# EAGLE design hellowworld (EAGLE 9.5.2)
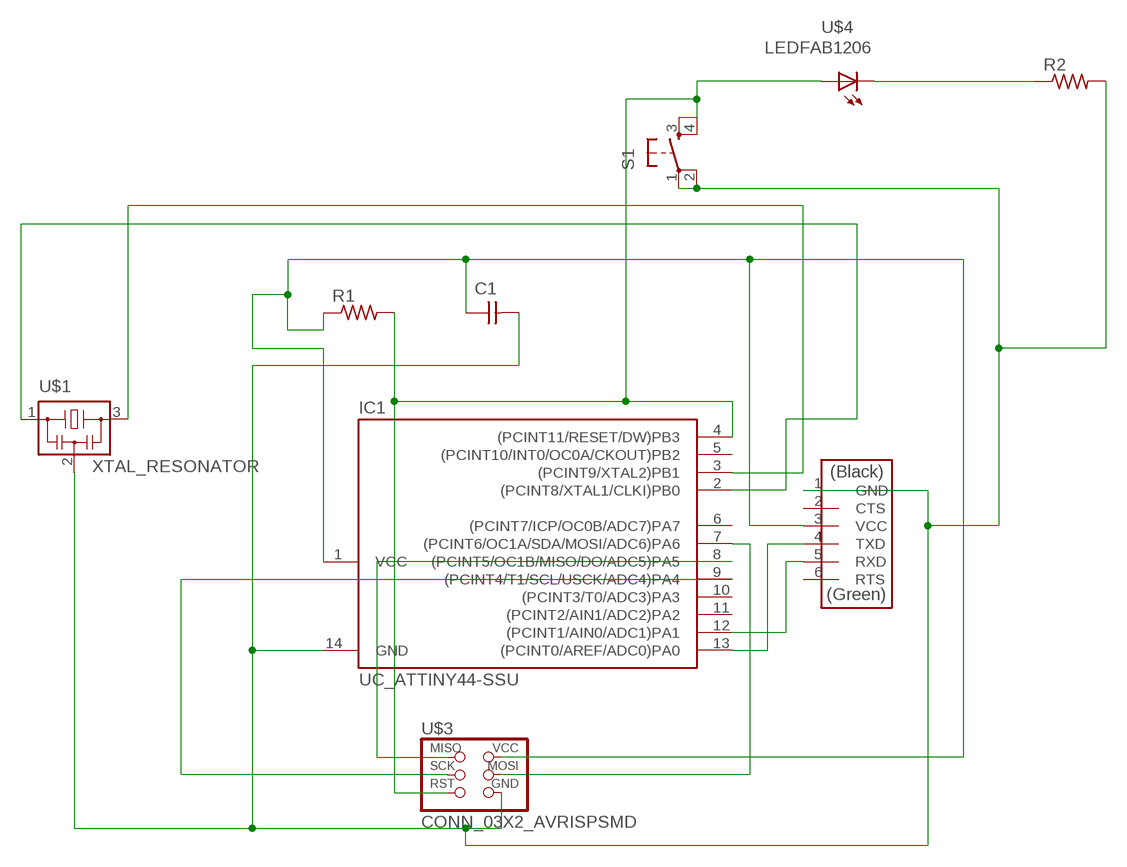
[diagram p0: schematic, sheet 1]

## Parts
C1  CAP_UNPOLARIZEDFAB  [C1206FAB]
IC1  UC_ATTINY44-SSU  [SOIC14]
R1  R1206FAB  [R1206FAB]
R2  R1206FAB  [R1206FAB]
S1  SW_SWITCH_TACTILE_6MM6MM_SWITCH  [6MM_SWITCH]
U$1  XTAL_RESONATOR  [EFOBM]
U$2  CONN_06_FTDI-SMD-HEADER  [1X06SMD]
U$3  CONN_03X2_AVRISPSMD  [2X03SMD]
U$4  LEDFAB1206  [LED1206FAB]

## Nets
N$1: IC1.13((PCINT0/AREF/ADC0)PA0) U$2.4(TXD)
N$2: C1.2 IC1.14(GND) R2.2 S1.1(P) S1.2(P1) U$1.2 U$2.1(GND) U$3.6(GND)
N$3: IC1.7((PCINT6/OC1A/SDA/MOSI/ADC6)PA6) U$3.4(MOSI)
N$4: IC1.8((PCINT5/OC1B/MISO/DO/ADC5)PA5) U$3.1(MISO)
N$5: IC1.9((PCINT4/T1/SCL/USCK/ADC4)PA4) U$3.3(SCK)
N$6: C1.1 IC1.1(VCC) R1.1 U$2.3(VCC) U$3.2(VCC)
N$7: IC1.2((PCINT8/XTAL1/CLKI)PB0) U$1.1
N$8: IC1.3((PCINT9/XTAL2)PB1) U$1.3
N$9: IC1.12((PCINT1/AIN0/ADC1)PA1) U$2.5(RXD)
N$10: R2.1 U$4.2(C)
N$11: IC1.4((PCINT11/RESET/DW)PB3) R1.2 S1.3(S) S1.4(S1) U$3.5(RST) U$4.1(A)
Unconnected: IC1.5((PCINT10/INT0/OC0A/CKOUT)PB2) IC1.6((PCINT7/ICP/OC0B/ADC7)PA7) IC1.10((PCINT3/T0/ADC3)PA3) IC1.11((PCINT2/AIN1/ADC2)PA2) U$2.2(CTS) U$2.6(RTS)

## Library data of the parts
C1 = eagle_fab:CAP_UNPOLARIZED
IC1 = eagle_fab:UC_ATTINY44
R1 R2 = eagle_fab:R: Resistor (US Symbol)
S1 = eagle_fab:SW_SWITCH_TACTILE_6MM: OMRON SWITCH
U$1 = eagle_fab:XTAL_RESONATOR
U$2 = eagle_fab:CONN_06_FTDI-SMD-HEADER
U$3 = eagle_fab:CONN_03X2_AVRISP
U$4 = eagle_fab:LED: LED

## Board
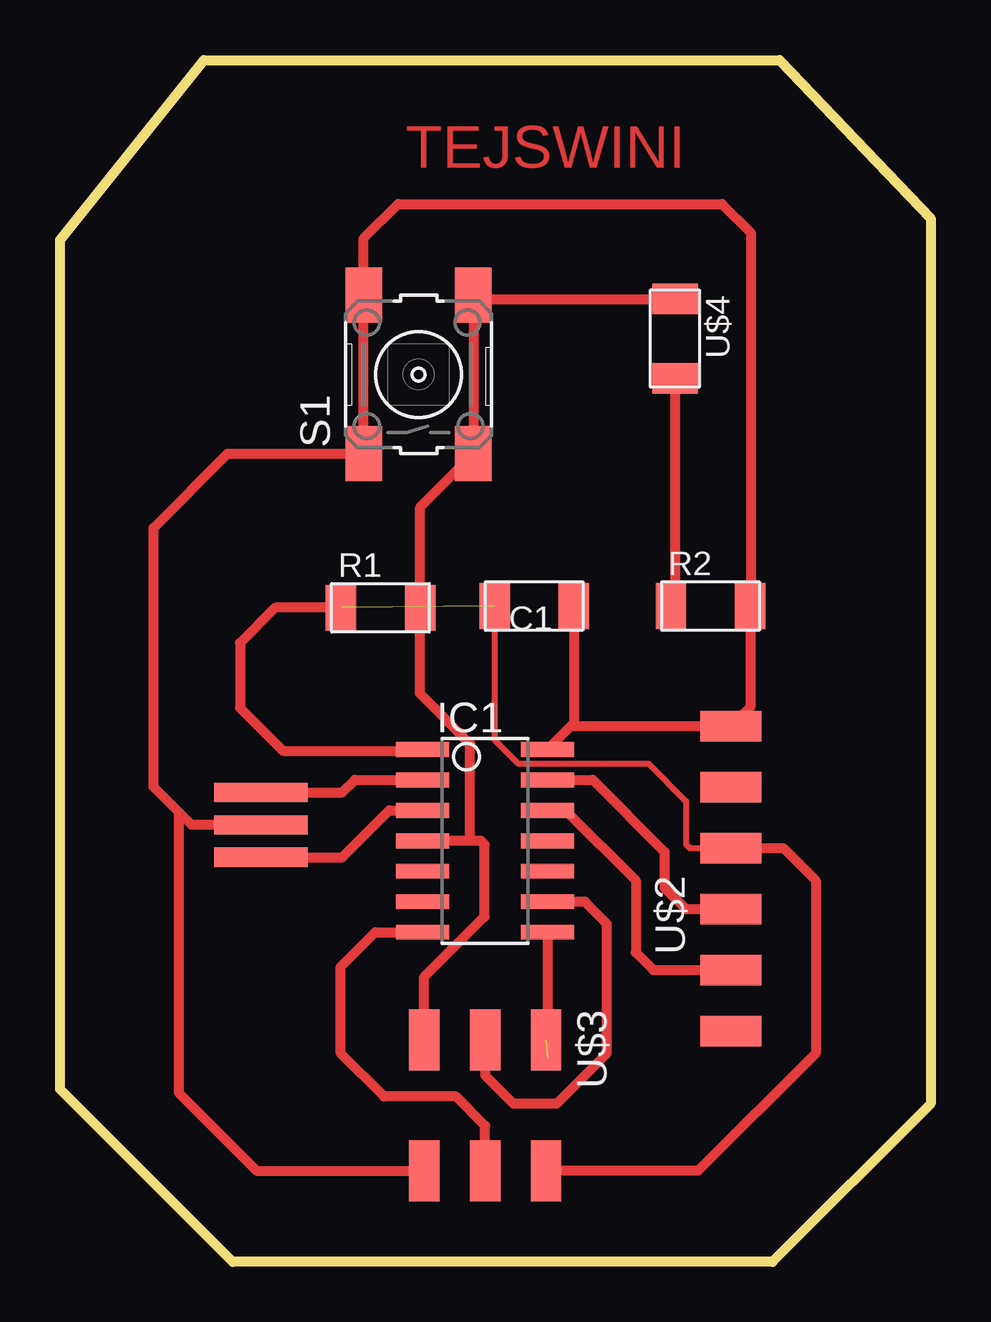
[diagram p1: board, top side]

Size 36.3 x 50.1 mm. Coordinates in mm from the lower left corner, seen from the top.
Outline: 6,50.1 30,50.1 36.3,43.5 36.3,6.6 29.7,0 7.2,0 0,7.2 0,42.6 6,50.1
Copper layers (1*16): Top 0.035mm / dielectric 1.5mm / Bottom 0.035mm
Design rules "default": minimum track width 6mil, minimum drill 0.35mm, track to track 6mil, track to pad 6mil, pad to pad 6mil, via to via 6mil, smd to smd 6mil, copper to edge 40mil, drill to drill 6mil, minimum pad ring 10mil, minimum via ring 8mil, stop-mask expansion 4mil, vias tented up to drill 0mil, thermal gap 10mil

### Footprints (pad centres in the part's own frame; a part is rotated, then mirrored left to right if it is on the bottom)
C1206FAB = smd 1.27 x 1.905: 1 -1.651,0; 2 1.651,0
SOIC14 = smd 0.61 x 2.21: 1 -3.81,-2.603; 2 -2.54,-2.603; 3 -1.27,-2.603; 4 0,-2.603; 5 1.27,-2.603; 6 2.54,-2.603; 7 3.81,-2.603; 8 3.81,2.603; 9 2.54,2.603; 10 1.27,2.603; 11 0,2.603; 12 -1.27,2.603; 13 -2.54,2.603; 14 -3.81,2.603
R1206FAB = smd 1.27 x 1.905: 1 -1.651,0; 2 1.651,0
6MM_SWITCH = smd 2.286 x 1.524: 1 -3.302,2.286; 2 3.302,2.286; 3 -3.302,-2.286; 4 3.302,-2.286
EFOBM = smd 0.8 x 3.9: 1 -1.35,0; 2 0,0; 3 1.35,0
1X06SMD = smd 2.54 x 1.27: 1 0,6.35; 2 0,3.81; 3 0,1.27; 4 0,-1.27; 5 0,-3.81; 6 0,-6.35
2X03SMD = smd 2.54 x 1.27: 1 -2.54,2.54; 2 2.92,2.54; 3 -2.54,0; 4 2.92,0; 5 -2.54,-2.54; 6 2.92,-2.54
LED1206FAB = smd 1.27 x 1.905: 1 -1.651,0; 2 1.651,0

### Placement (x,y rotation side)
C1  19.77,27.34 0 top
IC1  17.72,17.55 270 top
R1  13.36,27.27 0 top
R2  27.12,27.34 0 top
S1  14.95,36.99 90 top
U$1  8.37,18.22 270 top
U$2  27.97,15.98 0 top
U$3  17.72,6.72 270 top
U$4  25.64,38.49 270 top

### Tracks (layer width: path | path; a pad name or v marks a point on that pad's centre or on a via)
N$1
  Top 0.152: 27.97,15.02 U$2.4
  Top 0.406: 20.33,20.1 IC1.13 22.21,20.09 25.2,17.1 25.2,15.6 26.09,14.71 U$2.4
N$2
  Top 0.152: 21.42,28.07 C1.2 | 26.96,22.33 U$2.1
  Top 0.203: C1.2 21,27.76 | 28.14,22.5 U$2.1 | 12.66,33.96 S1.1 | 15.14,3.76 U$3.6
  Top 0.406: 19.6,21.36 IC1.14 | 21.46,27.3 C1.2 21.42,22.46 IC1.14 | S1.1 12.9,33.45 | S1.2 12.9,40.06 | IC1.14 21.29,22.33 U$2.1 28.77,23.13 R2.2 28.8,27.37 28.8,42.9 27.6,44.1 14.1,44.1 12.66,42.66 S1.2 | S1.1 12.66,39.9 | 12.66,39.9 S1.2 | 14.98,3.6 15.14,3.76 | 12.6,39.96 12.66,39.9 | U$1.2 5.48,18.22 4.95,18.75 | 4.95,18.75 3.9,19.8 3.9,30.6 6.99,33.69 S1.1 | 4.95,18.75 4.95,7.05 8.2,3.8 U$3.6
N$3
  Top 0.406: U$3.4 17.72,5.68 16.5,6.9 13.5,6.9 11.7,8.7 11.7,12.3 13.14,13.74 IC1.7
N$4  (1 unrouted)
  Top 0.152: IC1.8 20.26,13.68
  Top 0.406: 20.32,8.48 20.4,8.4 | IC1.8 20.32,9.32 U$3.1
N$5
  Top 0.406: 17.72,8.38 U$3.3 17.72,7.78 18.9,6.6 20.7,6.6 22.8,8.7 22.8,14.1 21.89,15.01 IC1.9
N$6  (1 unrouted)
  Top 0.152: U$3.2 20.64,4.18 | 15.18,21.36 IC1.1
  Top 0.203: 15.06,21.3 IC1.1
  Top 0.254: C1.1 18.12,21.76 19.1,20.78 24.52,20.78 26.1,19.2 26.1,17.4 26.25,17.25 U$2.3
  Top 0.406: U$2.3 28.12,17.1 27.9,17.1 | 15.12,21.3 15.18,21.36 | 20.36,3.9 U$3.2 26.6,3.8 31.5,8.7 31.5,15.9 30.15,17.25 U$2.3 | R1.1 8.97,27.27 7.5,25.8 7.5,23.1 9.3,21.3 15.06,21.3 | 28.95,17.25 U$2.3
N$7
  Top 0.152: U$1.1 8.45,19.49
  Top 0.406: 8.44,19.5 U$1.1 11.77,19.57 12.3,20.1 15.11,20.1 IC1.2
N$8
  Top 0.203: 9.67,16.87 U$1.3
  Top 0.406: U$1.3 11.77,16.87 13.72,18.82 IC1.3
N$9
  Top 0.152: 27.97,12.48 U$2.5 27.92,12.53
  Top 0.406: IC1.12 21.08,18.82 24,15.9 24,12.9 24.73,12.17 U$2.5
N$10
  Top 0.406: U$4.2 25.64,27.51 R2.1
N$11
  Top 0.152: U$4.1 25.35,39.85
  Top 0.203: S1.3 16.73,33.18 | S1.4 17.33,40.2
  Top 0.406: S1.3 17.49,33.43 | S1.3 17.4,33.69 | 17.4,33.69 17.61,33.69 | U$3.5 15.18,11.88 17.7,14.4 17.7,17.4 17.55,17.55 17.1,17.55 | 17.1,17.55 IC1.4 | S1.3 15.01,31.46 R1.2 15,27.26 15,23.7 17.1,21.6 17.1,17.55 | 17.4,33.69 17.24,33.85 S1.4 17.39,40.14 U$4.1

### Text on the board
Top: TEJSWINI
